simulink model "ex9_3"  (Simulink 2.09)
settings: Solver=ode45  StartTime=0.0  StopTime=1000.0  MaxStep=.1  RelTol=1e-3  AbsTol=1e-6

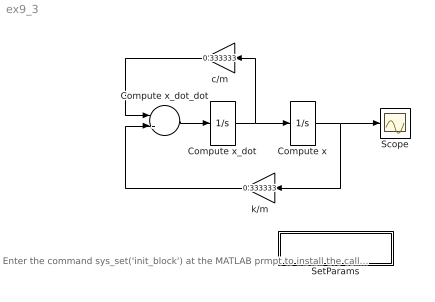
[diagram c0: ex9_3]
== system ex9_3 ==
  note: Enter the command sys_set('init_block') at the MATLAB prmpt to install the callback.
  Compute x : Integrator  ExternalReset=none  InitialConditionSource=internal  InitialCondition=0  LimitOutput=off  UpperSaturationLimit=inf  LowerSaturationLimit=-inf  ShowSaturationPort=off  ShowStatePort=off  AbsoluteTolerance=auto
  Compute x_dot : Integrator  ExternalReset=none  InitialConditionSource=internal  InitialCondition=1  LimitOutput=off  UpperSaturationLimit=inf  LowerSaturationLimit=-inf  ShowSaturationPort=off  ShowStatePort=off  AbsoluteTolerance=auto
  Compute x_dot_dot : Sum  Inputs=--
  Scope : Scope
  SetParams : Subsystem  mask{m=3.000000, c=1.000000, k=1.000000}
      mask prompts: m "Mass"; c "Damping coefficient"; k "Spring constant"
      mask help: This masked subsystem supports the spring-mass user interface. The dialog fiellds are not available to the user due to the use of the OperFcn callback.
  c/m : Gain  Orientation=left  Gain=0.333333
  k/m : Gain  Orientation=left  Gain=0.333333
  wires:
  Compute x_dot_dot/1 -> Compute x_dot/1
  c/m/1 -> Compute x_dot_dot/1
  Compute x_dot/1 -> Compute x/1, c/m/1
  k/m/1 -> Compute x_dot_dot/2
  Compute x/1 -> k/m/1, Scope/1

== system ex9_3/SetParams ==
  note: This is an empty subsystem. The purpose of the subsystem is to provide a means to open the sys_set user interface.
